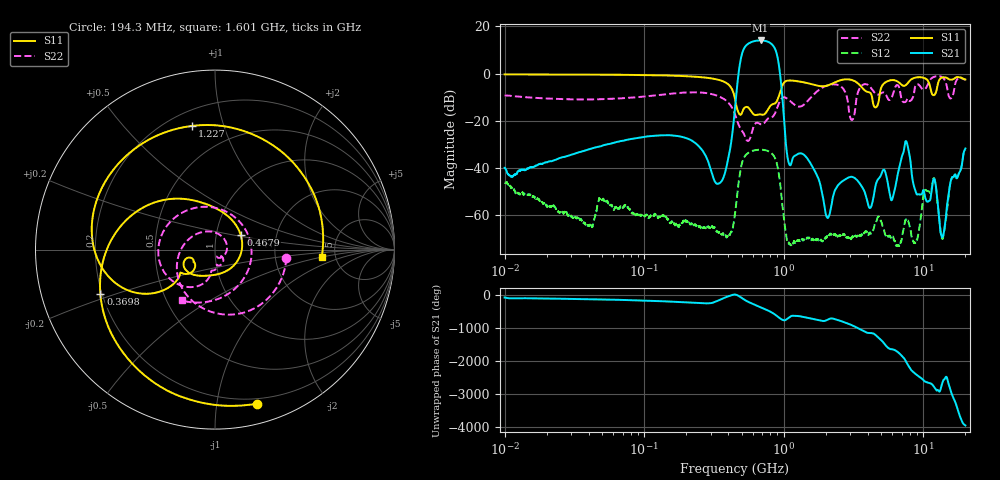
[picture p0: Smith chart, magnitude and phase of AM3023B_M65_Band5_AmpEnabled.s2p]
!Agilent Technologies,E8364B,MY43040894,A.07.50.67
!Agilent E8364B: A.07.50.67
!Date: Tuesday, October 27, 2020 10:53:21
!Correction: S11(Full 2 Port(1,2))
!S21(Full 2 Port(1,2))
!S12(Full 2 Port(1,2))
!S22(Full 2 Port(1,2))
!S2P File: Measurements: S11, S21, S12, S22:Log Frequency Sweep
# Hz S  dB  R 50
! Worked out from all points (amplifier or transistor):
!   3201 points, 10 MHz to 20 GHz, reference 50 ohm
!   highest |S21| = 14.1 dB at 682.6 MHz (marker M1)
!   |S21| within 3 dB of that: 523.5 MHz to 856.2 MHz (332.7 MHz wide, 48.2 % of centre)
!   unconditionally stable (mu >= 1): start of sweep to end of sweep
!   at 35.47 MHz: K = 2015.22, MAG = -21.7 dB, |S12| = -61.7 dB
!   at 447.2 MHz: K = 2204.34, MAG = -14.1 dB, |S12| = -59.3 dB
!   at 20 GHz: K = 150.50, MAG = -24.5 dB, |S12| = -32.2 dB
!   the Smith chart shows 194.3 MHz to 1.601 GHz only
!   S11 on the Smith chart (normalised r, x): 194.3 MHz: 0.16, -1.30; 369.8 MHz: 0.19, -0.18; 467.9 MHz: 1.31, +0.22; 1.227 GHz: 0.29, +0.79; 1.601 GHz: 3.89, -0.49
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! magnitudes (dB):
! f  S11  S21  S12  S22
! 10 MHz  -0.3  -39.8  -46.1  -9.2
! 35.55 MHz  -0.4  -33.0  -62.0  -10.9
! 126.1 MHz  -0.7  -26.2  -61.1  -9.1
! 194.3 MHz  -1.0  -27.0  -62.4  -8.0
! 369.8 MHz  -3.3  -43.9  -67.9  -10.6
! 447.2 MHz  -10.7  -14.5  -59.3  -17.2
! 467.9 MHz  -15.7  -2.8  -49.4  -20.6
! 682.6 MHz  -17.2  14.1  -32.2  -21.4
! 880.1 MHz  -12.2  9.4  -36.8  -15.8
! 1.072 GHz  -2.9  -36.4  -71.7  -10.8
! 1.227 GHz  -3.1  -34.4  -70.9  -13.6
! 1.59 GHz  -4.4  -39.0  -70.3  -9.6
! 1.601 GHz  -4.5  -39.3  -70.2  -9.4
! 2.06 GHz  -5.0  -61.0  -68.9  -4.9
! 2.886 GHz  -2.4  -44.0  -69.2  -12.3
! 4.543 GHz  -14.3  -47.4  -63.0  -8.5
! 5.639 GHz  -3.0  -48.3  -68.5  -11.0
! 7.588 GHz  -4.5  -29.0  -61.5  -11.3
! 8.961 GHz  -1.5  -51.1  -70.4  -4.4
! 11.92 GHz  -9.1  -44.6  -44.2  -1.3
! 13.71 GHz  -1.5  -69.2  -70.0  -1.5
! 20 GHz  -2.4  -31.6  -32.2  -2.6
